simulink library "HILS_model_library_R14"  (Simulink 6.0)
undefined symbols (not defined in the file or in its folder): hilsmdl
libraries: simulink x47, simulink_extras x9, HILS_model_library x3
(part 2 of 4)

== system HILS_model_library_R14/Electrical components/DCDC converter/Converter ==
  ctrl : Inport
  elec in [V] : Inport  Port=2
  elec fb in [A] : Inport  Port=3
  Bus Creator : BusCreator  Inputs=1
  Bus Creator1 : BusCreator  Inputs=2
  Bus Creator5 : BusCreator  Inputs=1
  Bus Selector1 : BusSelector  OutputSignals=phys_current_A
  Bus Selector2 : BusSelector  OutputSignals=Dcdc_ctrl_Rt
  Bus Selector5 : BusSelector  OutputSignals=phys_voltage_V
  Gain : Gain
  Gain1 : Gain
  Memory : Memory  Orientation=left
  Product : Product
  Product1 : Product  Inputs=3
  Sensor : Outport
  elec out [V] : Outport  Port=2
  elec fb out [A] : Outport  Port=3
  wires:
  Bus Creator1/1 -> Sensor/1
  Bus Creator/1 -> elec out [V]/1
  elec in [V]/1 -> Bus Selector5/1
  Bus Creator5/1 -> elec fb out [A]/1
  elec fb in [A]/1 -> Bus Selector1/1
  ctrl/1 -> Bus Selector2/1
  Product/1 -> Bus Creator/1, Gain/1  "phys_voltage_V"
  Product1/1 -> Memory/1, Bus Creator5/1  "phys_current_A"
  Bus Selector1/1 -> Product1/2  "<phys_current_A>"
  Bus Selector5/1 -> Gain1/1, Product/2  "<phys_voltage_V>"
  Bus Selector2/1 -> Product1/1, Product/1  "<Dcdc_ctrl_Rt>"
  Gain/1 -> Bus Creator1/2  "voltage_out"
  Gain1/1 -> Bus Creator1/1  "voltage_in"
  ? -> Product1/3
  Memory/1 -> ?

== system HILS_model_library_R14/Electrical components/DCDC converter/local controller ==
  cmd : Inport
  sensor in : Inport  Port=2
  Bus Creator1 : BusCreator  Inputs=1
  Bus Creator2 : BusCreator  Inputs=1
  Bus Selector1 : BusSelector  OutputSignals=Dcdc_uReq_V
  Bus Selector2 : BusSelector  OutputSignals=voltage_in,voltage_out
  Gain : Gain
  Product : Product  Inputs=*/
  sensor out : Outport
  ctrl : Outport  Port=2
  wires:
  Bus Creator1/1 -> ctrl/1
  sensor in/1 -> Bus Selector2/1
  cmd/1 -> Bus Selector1/1
  Bus Creator2/1 -> sensor out/1  "Dcdc"
  Bus Selector2/1 -> Product/2  "<voltage_in>"
  Bus Selector2/2 -> Gain/1  "<voltage_out>"
  Gain/1 -> Bus Creator2/1  "Dcdc_uAct_V"
  Bus Selector1/1 -> Product/1  "<Dcdc_uReq_V>"
  Product/1 -> Bus Creator1/1  "Dcdc_ctrl_Rt"

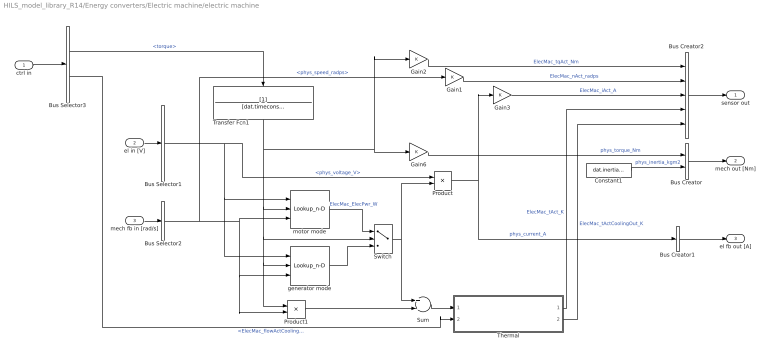
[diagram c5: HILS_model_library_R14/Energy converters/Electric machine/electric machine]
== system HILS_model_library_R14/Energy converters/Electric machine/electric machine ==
  ctrl in : Inport
  el in [V] : Inport  Port=2
  mech fb in [rad/s] : Inport  Port=3
  Bus Creator : BusCreator  Inputs=2
  Bus Creator1 : BusCreator  Inputs=1
  Bus Creator2 : BusCreator  Inputs=5
  Bus Selector1 : BusSelector  OutputSignals=phys_voltage_V
  Bus Selector2 : BusSelector  OutputSignals=phys_speed_radps
  Bus Selector3 : BusSelector  OutputSignals=torque,ElecMac_flowActCooling_kgps
  Constant1 : Constant  Value=dat.inertia.value
  Gain{1..3,6} (4 alike) : Gain
  Product : Product  Inputs=/*
  Product1 : Product  Inputs=**
  Sum : Sum  Inputs=+-
  Switch : Switch
  Thermal : Subsystem
  Transfer Fcn1 : TransferFcn  Orientation=down  Denominator=[dat.timeconstant.value 1]
  generator mode : Lookup_n-D  NumberOfTableDimensions=3  BreakpointsForDimension1=dat.elecpowmap.generator.voltage.vec  BreakpointsForDimension2=dat.elecpowmap.generator.torque.vec  BreakpointsForDimension3=dat.elecpowmap.generator.speed.vec  Table=dat.elecpowmap.generator.elecpow.map  ExtrapMethod=None - Clip
  motor mode : Lookup_n-D  NumberOfTableDimensions=3  BreakpointsForDimension1=dat.elecpowmap.motor.voltage.vec  BreakpointsForDimension2=dat.elecpowmap.motor.torque.vec  BreakpointsForDimension3=dat.elecpowmap.motor.speed.vec  Table=dat.elecpowmap.motor.elecpow.map  ExtrapMethod=None - Clip
  sensor out : Outport
  mech out [Nm] : Outport  Port=2
  el fb out [A] : Outport  Port=3
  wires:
  Sum/1 -> Thermal/1(Total power loss)
  Product1/1 -> Sum/2
  Thermal/1(Machine temperature[K]) -> Bus Creator2/4  "ElecMac_tAct_K"
  Gain6/1 -> Bus Creator/1  "phys_torque_Nm"
  Gain2/1 -> Bus Creator2/1  "ElecMac_tqAct_Nm"
  Gain1/1 -> Bus Creator2/2  "ElecMac_nAct_radps"
  Gain3/1 -> Bus Creator2/3  "ElecMac_iAct_A"
  Product/1 -> Gain3/1, Bus Creator1/1  "phys_current_A"
  Bus Selector3/1 -> Transfer Fcn1/1  "<torque>"
  Constant1/1 -> Bus Creator/2  "phys_inertia_kgm2"
  Bus Creator2/1 -> sensor out/1
  Bus Selector2/1 -> Gain1/1, Product1/2, generator mode/3, motor mode/3  "<phys_speed_radps>"
  ctrl in/1 -> Bus Selector3/1
  mech fb in [rad/s]/1 -> Bus Selector2/1
  el in [V]/1 -> Bus Selector1/1
  Bus Creator/1 -> mech out [Nm]/1
  Bus Creator1/1 -> el fb out [A]/1
  motor mode/1 -> Switch/1  "ElecMac_ElecPwr_W"
  generator mode/1 -> Switch/3
  Switch/1 -> Product/2, Sum/1
  Bus Selector1/1 -> Product/1, motor mode/1, generator mode/1  "<phys_voltage_V>"
  Transfer Fcn1/1 -> Gain2/1, Gain6/1, Product1/1, generator mode/2, Switch/2, motor mode/2
  Bus Selector3/2 -> Thermal/2(Massflow cooling fluid)  "<ElecMac_flowActCooling_kgps>"
  Thermal/2(Fluid outlet temperature[K]) -> Bus Creator2/5  "ElecMac_tActCoolingOut_K"

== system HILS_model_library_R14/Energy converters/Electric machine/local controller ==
  cmd in : Inport
  sensor in : Inport  Port=2
  Bus Creator2 : BusCreator
  Bus Selector1 : BusSelector  OutputSignals=ElecMac_nReq_radps,ElecMac_flgReqSwitch_B,ElecMac_tqReq_Nm,ElecMac_flowActCooling_kgps
  Bus Selector3 : BusSelector  OutputSignals=ElecMac_tqAct_Nm,ElecMac_nAct_radps,ElecMac_iAct_A,ElecMac_tAct_K
  Bus Creator : BusCreator  Inputs=2
  Compare To Zero : simulink/Logic and Bit Operations/Compare To Zero  relop=>  LogicOutDataTypeMode=uint8  ZeroCross=off
  Max torque : Lookup  InputValues=dat.maxtorque.speed.vec  OutputValues=dat.maxtorque.torque.vec  LookUpMeth=Interpolation-Use End Values
  Min torque : Lookup  InputValues=dat.mintorque.speed.vec  OutputValues=dat.mintorque.torque.vec  LookUpMeth=Interpolation-Use End Values
  PI controller : Subsystem
  Product : Product
  Saturation Dynamic : simulink/Discontinuities/Saturation Dynamic  OutDataType=fixdt(1, 16)  OutScaling=2^-10  DoSatur=off
  Switch1 : Switch  Threshold=0.5
  Switch2 : Switch  Threshold=0.5
  sensor out : Outport
  ctrl out : Outport  Port=2
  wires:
  Bus Selector3/4 -> Bus Creator2/4  "<ElecMac_tAct_K>"
  Compare To Zero/1 -> Product/1
  Product/1 -> Switch2/1
  PI controller/1(Ctrl signal) -> Product/2
  Min torque/1 -> Saturation Dynamic/3
  Max torque/1 -> Saturation Dynamic/1
  Switch2/1 -> Saturation Dynamic/2
  Switch1/1 -> PI controller/1(RefSpeed), Switch2/3
  Saturation Dynamic/1 -> Bus Creator/1  "torque"
  Bus Creator/1 -> ctrl out/1
  Bus Selector3/3 -> Bus Creator2/3  "<ElecMac_iAct_A>"
  Bus Selector3/2 -> Min torque/1, Max torque/1, Bus Creator2/2, PI controller/2(ActSpeed)  "<ElecMac_nAct_radps>"
  Bus Selector3/1 -> Bus Creator2/1  "<ElecMac_tqAct_Nm>"
  sensor in/1 -> Bus Selector3/1
  Bus Creator2/1 -> sensor out/1  "ElectricMachine"
  Bus Selector1/3 -> Switch1/3  "<ElecMac_tqReq_Nm>"
  Bus Selector1/2 -> Switch1/2, Switch2/2, PI controller/3(Reset)  "<ElecMac_flgReqSwitch_B>"
  Bus Selector1/1 -> Switch1/1, Compare To Zero/1  "<ElecMac_nReq_radps>"
  cmd in/1 -> Bus Selector1/1
  Bus Selector1/4 -> Bus Creator/2  "<ElecMac_flowActCooling_kgps>"

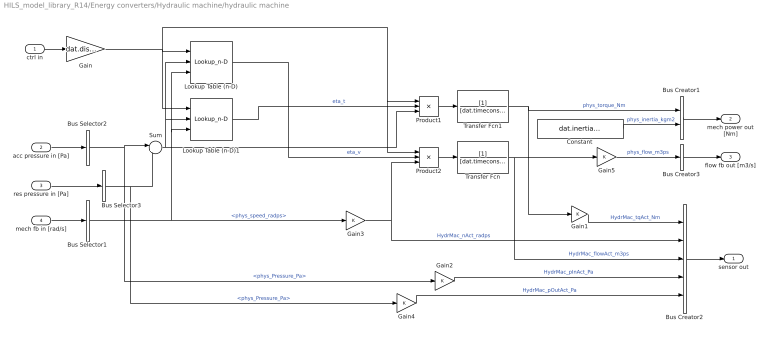
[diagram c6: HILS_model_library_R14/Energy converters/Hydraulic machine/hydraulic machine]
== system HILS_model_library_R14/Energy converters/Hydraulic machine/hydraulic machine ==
  ctrl in : Inport
  acc pressure in [Pa] : Inport  Port=2
  res pressure in [Pa] : Inport  Port=3
  mech fb in [rad/s] : Inport  Port=4
  Bus Creator1 : BusCreator  Inputs=2
  Bus Creator2 : BusCreator  Inputs=5
  Bus Creator3 : BusCreator  Inputs=1
  Bus Selector1 : BusSelector  OutputSignals=phys_speed_radps
  Bus Selector2 : BusSelector  OutputSignals=phys_Pressure_Pa
  Bus Selector3 : BusSelector  OutputSignals=phys_Pressure_Pa
  Constant : Constant  Value=dat.inertia.value
  Gain : Gain  Gain=dat.displacement.value
  Gain{1..5} (5 alike) : Gain
  Lookup Table (n-D) : Lookup_n-D  NumberOfTableDimensions=3  BreakpointsForDimension1=dat.volefficiency.x.vec  BreakpointsForDimension2=dat.volefficiency.pressure.vec  BreakpointsForDimension3=dat.volefficiency.speed.vec  BreakpointsForDimension4=hydraulic_speed_vec_radps  Table=dat.volefficiency.efficiency.map  ExtrapMethod=None - Clip
  Lookup Table (n-D)1 : Lookup_n-D  NumberOfTableDimensions=3  BreakpointsForDimension1=dat.mechefficiency.x.vec  BreakpointsForDimension2=dat.mechefficiency.pressure.vec  BreakpointsForDimension3=dat.mechefficiency.speed.vec  BreakpointsForDimension4=hydraulic_speed_vec_radps  Table=dat.mechefficiency.efficiency.map  ExtrapMethod=None - Clip
  Product1 : Product  Inputs=3
  Product2 : Product  Inputs=3
  Sum : Sum  Inputs=|+-
  Transfer Fcn : TransferFcn  Denominator=[dat.timeconstant.value 1]
  Transfer Fcn1 : TransferFcn  Denominator=[dat.timeconstant.value 1]
  sensor out : Outport
  mech power out [Nm] : Outport  Port=2
  flow fb out [m3/s] : Outport  Port=3
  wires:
  ctrl in/1 -> Gain/1
  Product1/1 -> Transfer Fcn1/1
  Product2/1 -> Transfer Fcn/1
  Gain/1 -> Product1/1, Product2/1, Lookup Table (n-D)/1, Lookup Table (n-D)1/1
  Transfer Fcn/1 -> Bus Creator2/3, Gain5/1  "HydrMac_flowAct_m3ps"
  Transfer Fcn1/1 -> Gain1/1, Bus Creator1/1  "phys_torque_Nm"
  acc pressure in [Pa]/1 -> Bus Selector2/1
  res pressure in [Pa]/1 -> Bus Selector3/1
  Sum/1 -> Product1/3, Lookup Table (n-D)/2, Lookup Table (n-D)1/2
  Bus Creator2/1 -> sensor out/1
  Gain3/1 -> Bus Creator2/2, Product2/3  "HydrMac_nAct_radps"
  Constant/1 -> Bus Creator1/2  "phys_inertia_kgm2"
  Bus Creator1/1 -> mech power out [Nm]/1
  mech fb in [rad/s]/1 -> Bus Selector1/1
  Bus Selector1/1 -> Gain3/1, Lookup Table (n-D)/3, Lookup Table (n-D)1/3  "<phys_speed_radps>"
  Lookup Table (n-D)1/1 -> Product1/2  "eta_t"
  Bus Creator3/1 -> flow fb out [m3/s]/1
  Gain1/1 -> Bus Creator2/1  "HydrMac_tqAct_Nm"
  Bus Selector2/1 -> Sum/1, Gain2/1  "<phys_Pressure_Pa>"
  Bus Selector3/1 -> Gain4/1, Sum/2  "<phys_Pressure_Pa>"
  Gain2/1 -> Bus Creator2/4  "HydrMac_pInAct_Pa"
  Gain4/1 -> Bus Creator2/5  "HydrMac_pOutAct_Pa"
  Gain5/1 -> Bus Creator3/1  "phys_flow_m3ps"
  Lookup Table (n-D)/1 -> Product2/2  "eta_v"

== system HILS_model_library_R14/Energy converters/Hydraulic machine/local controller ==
  cmd in : Inport
  sensor in : Inport  Port=2
  Bus Creator1 : BusCreator  Inputs=1
  Bus Creator2 : BusCreator  Inputs=5
  Bus Selector1 : BusSelector  OutputSignals=HydrMac_nReq_radps,HydrMac_flgRegSwitch_B,HydrMac_tqReg_Nm
  Bus Selector3 : BusSelector  OutputSignals=HydrMac_tqAct_Nm,HydrMac_nAct_radps,HydrMac_flowAct_m3ps,HydrMac_pInAct_Pa,HydrMac_pOutAct_Pa
  PI controller : Subsystem
  Saturation : Saturate  UpperLimit=1  LowerLimit=-1
  Switch1 : Switch  Threshold=0.5
  Switch2 : Switch  Threshold=0.5
  sensor out : Outport
  ctrl out : Outport  Port=2
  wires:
  cmd in/1 -> Bus Selector1/1
  Bus Selector1/1 -> Switch1/1  "<HydrMac_nReq_radps>"
  Bus Selector1/2 -> Switch2/2, PI controller/3(Reset), Switch1/2  "<HydrMac_flgRegSwitch_B>"
  Bus Selector1/3 -> Switch1/3  "<HydrMac_tqReg_Nm>"
  Bus Creator2/1 -> sensor out/1  "HydrMac"
  sensor in/1 -> Bus Selector3/1
  Bus Selector3/2 -> Bus Creator2/2, Switch2/1  "<HydrMac_nAct_radps>"
  Bus Creator1/1 -> ctrl out/1
  Switch1/1 -> PI controller/1(Ref)
  Bus Selector3/1 -> Bus Creator2/1, Switch2/3  "<HydrMac_tqAct_Nm>"
  Switch2/1 -> PI controller/2(Act)
  PI controller/1(Ctrl signal) -> Saturation/1
  Saturation/1 -> Bus Creator1/1
  Bus Selector3/3 -> Bus Creator2/3  "<HydrMac_flowAct_m3ps>"
  Bus Selector3/4 -> Bus Creator2/4  "<HydrMac_pInAct_Pa>"
  Bus Selector3/5 -> Bus Creator2/5  "<HydrMac_pOutAct_Pa>"

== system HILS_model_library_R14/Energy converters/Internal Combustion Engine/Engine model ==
  ctrl in : Inport
  mech fb in [rad/s] : Inport  Port=2
  Bus Creator : BusCreator  Inputs=2
  Bus Creator2 : BusCreator  Inputs=5
  Bus Selector2 : BusSelector  OutputSignals=phys_speed_radps
  Bus Selector3 : BusSelector  OutputSignals=Eng_tqIndReq_Nm,Eng_flgFuelCut_B,Eng_flgOnOff_B,Eng_flgStrtReq_B,Eng_flgExhaustBrake
  Constant1 : Constant  Value=dat.inertia.value
  Engine brake : Lookup  InputValues=dat.exhaustbrake.speed.vec  OutputValues=dat.exhaustbrake.brake.vec  LookUpMeth=Interpolation-Use End Values
  Friction map : Lookup  InputValues=dat.friction.speed.vec  OutputValues=dat.friction.friction.vec  LookUpMeth=Interpolation-Use End Values
  Memory : Memory
  Product : Product
  Product1 : Product  Inputs=3
  Sum1 : Sum
  Sum2 : Sum
  Thermal model ICE : Subsystem
  Torque model1 : Subsystem
  radps2rpm1 : Gain
  radps2rpm2 : Gain
  sensor out : Outport
  mech power out [Nm] : Outport  Port=2
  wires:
  Bus Selector3/4 -> Torque model1/3(starter motor)  "<Eng_flgStrtReq_B>"
  Bus Selector3/3 -> Product1/3  "<Eng_flgOnOff_B>"
  Memory/1 -> Thermal model ICE/2(Eng speed), radps2rpm2/1, Torque model1/2(speed rps), Engine brake/1, Friction map/1
  Bus Creator/1 -> mech power out [Nm]/1
  mech fb in [rad/s]/1 -> Bus Selector2/1
  ctrl in/1 -> Bus Selector3/1
  Bus Selector2/1 -> Memory/1  "<phys_speed_radps>"
  Bus Creator2/1 -> sensor out/1
  Constant1/1 -> Bus Creator/2  "phys_inertia_kgm2"
  Friction map/1 -> Sum2/2  "Eng_tqFrictionAct_Nm"
  Engine brake/1 -> Product/2
  Product/1 -> Sum1/2  "Eng_tqExhaustBrakeAct_Nm"
  Bus Selector3/1 -> Product1/1  "<Eng_tqIndReq_Nm>"
  Bus Selector3/5 -> Product/1  "<Eng_flgExhaustBrake>"
  radps2rpm1/1 -> Bus Creator2/1  "Eng_tqCrkSftAct_Nm"
  radps2rpm2/1 -> Bus Creator2/4  "Eng_nAct_radps"
  Sum1/1 -> Thermal model ICE/1(Torque ICE), radps2rpm1/1, Bus Creator/1  "phys_torque_Nm"
  Thermal model ICE/2(temperature oil [K]) -> Bus Creator2/3  "Eng_tOilAct_K"
  Thermal model ICE/1(temperature cooling fluid [K]) -> Bus Creator2/2  "Eng_tCoolantAct_K"
  Bus Selector3/2 -> Product1/2  "<Eng_flgFuelCut_B>"
  Product1/1 -> Bus Creator2/5, Torque model1/1(Torque in)  "Eng_tqIndAct_Nm"
  Torque model1/1(Torque out) -> Sum2/1
  Sum2/1 -> Sum1/1

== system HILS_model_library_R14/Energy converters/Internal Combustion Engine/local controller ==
  cmd in : Inport
  sensor in : Inport  Port=2
  Bus Creator1 : BusCreator  Inputs=5
  Bus Creator2 : BusCreator
  Bus Selector1 : BusSelector  OutputSignals=Eng_nReq_radps,Eng_flgReqSwitch_B,Eng_tqReq_Nm,Eng_flgFuelCut_B,Eng_flgExhaustBrake,Eng_flgOnOff_B,Eng_flgStrtReq_B
  Bus Selector3 : BusSelector  OutputSignals=Eng_nAct_radps,Eng_tqCrkSftAct_Nm,Eng_tqIndAct_Nm,Eng_tOilAct_K
  Speed controller : Subsystem
  Switch3 : Switch  Threshold=0.5
  Torque Limit : Subsystem
  Torque controller : Subsystem
  sensor : Outport
  ctrl out : Outport  Port=2
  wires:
  Bus Selector1/7 -> Bus Creator1/5  "<Eng_flgStrtReq_B>"
  Bus Selector1/6 -> Bus Creator1/4  "<Eng_flgOnOff_B>"
  cmd in/1 -> Bus Selector1/1
  Bus Selector1/1 -> Speed controller/1(RefSpeed)  "<Eng_nReq_radps>"
  Bus Selector1/2 -> Speed controller/3(Reset), Switch3/2  "<Eng_flgReqSwitch_B>"
  Bus Selector1/3 -> Torque controller/1(RefTorque)  "<Eng_tqReq_Nm>"
  Bus Creator2/1 -> sensor/1  "Engine"
  sensor in/1 -> Bus Selector3/1
  Bus Selector3/1 -> Torque controller/2(ActSpeed), Speed controller/2(ActSpeed), Torque Limit/2(ActSpeed), Bus Creator2/1  "<Eng_nAct_radps>"
  Bus Selector3/2 -> Bus Creator2/2  "<Eng_tqCrkSftAct_Nm>"
  Bus Creator1/1 -> ctrl out/1
  Speed controller/1(ctrl signal) -> Switch3/1
  Torque Limit/1(LimitTorqueDemand) -> Bus Creator1/1
  Switch3/1 -> Torque Limit/1(TorqueDemand)
  Torque controller/1(TotalTorqueRef) -> Switch3/3
  Bus Selector3/3 -> Bus Creator2/3  "<Eng_tqIndAct_Nm>"
  Bus Selector3/4 -> Bus Creator2/4  "<Eng_tOilAct_K>"
  Bus Selector1/5 -> Bus Creator1/3  "<Eng_flgExhaustBrake>"
  Bus Selector1/4 -> Bus Creator1/2  "<Eng_flgFuelCut_B>"

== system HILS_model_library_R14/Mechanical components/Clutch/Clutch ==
  ctrl : Inport
  mech in [Nm] : Inport  Port=2
  mech fb in [rad/s] : Inport  Port=3
  Bus Creator : BusCreator  Inputs=2
  Bus Creator1 : BusCreator  Inputs=1
  Bus Creator5 : BusCreator  Inputs=1
  Bus Selector1 : BusSelector  OutputSignals=phys_speed_radps
  Bus Selector2 : BusSelector  OutputSignals=Clu_ratReq_Rt
  Bus Selector5 : BusSelector  OutputSignals=phys_torque_Nm,phys_inertia_kgm2
  Clutch max  torque [Nm] : Constant  Value=dat.maxtorque.value
  Clutch1 : Subsystem
  Data Type Conversion : DataTypeConversion
  Product : Product
  Saturation : Saturate  UpperLimit=1  LowerLimit=0
  Transfer Fcn : TransferFcn  Denominator=[dat.actuator.timeconstant.value 1]
  sensor out : Outport
  mech out [Nm] : Outport  Port=2
  mech fb out [rad/s] : Outport  Port=3
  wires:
  Transfer Fcn/1 -> Clutch1/1(T_reqClu)
  Product/1 -> Transfer Fcn/1
  Saturation/1 -> Product/1
  Clutch max  torque [Nm]/1 -> Clutch1/5(Maxtorque), Product/2
  Bus Selector2/1 -> Saturation/1  "<Clu_ratReq_Rt>"
  Bus Selector1/1 -> Clutch1/4(w_down)  "<phys_speed_radps>"
  Clutch1/3(w_up) -> Bus Creator5/1  "phys_speed_radps"
  Clutch1/4(B_cluLock) -> Data Type Conversion/1
  Clutch1/1(T_out) -> Bus Creator/1  "phys_torque_Nm"
  ctrl/1 -> Bus Selector2/1
  Bus Creator1/1 -> sensor out/1  "Clutch"
  Bus Selector5/2 -> Clutch1/3(J_in)  "<phys_inertia_kgm2>"
  Bus Selector5/1 -> Clutch1/2(T_in)  "<phys_torque_Nm>"
  Data Type Conversion/1 -> Bus Creator1/1  "Clu_flgConnected_B"
  mech fb in [rad/s]/1 -> Bus Selector1/1
  Bus Creator5/1 -> mech fb out [rad/s]/1
  mech in [Nm]/1 -> Bus Selector5/1
  Bus Creator/1 -> mech out [Nm]/1
  Clutch1/2(J_out) -> Bus Creator/2  "phys_inertia_kgm2"

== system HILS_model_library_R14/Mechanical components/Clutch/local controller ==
  cmd in : Inport
  sensor in : Inport  Port=2
  sensor : Outport
  ctrl : Outport  Port=2
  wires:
  cmd in/1 -> ctrl/1
  sensor in/1 -> sensor/1

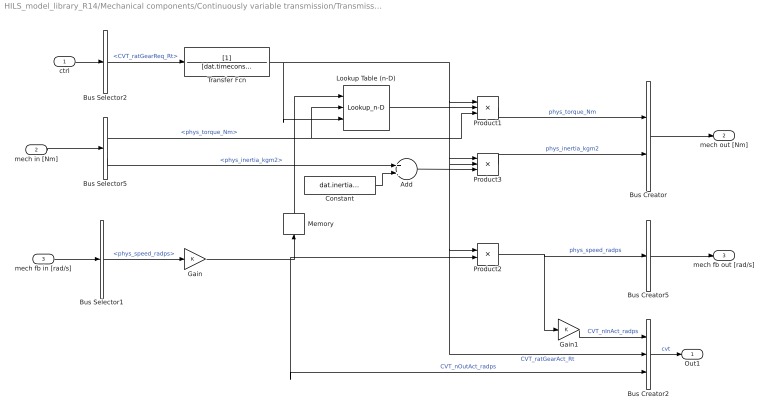
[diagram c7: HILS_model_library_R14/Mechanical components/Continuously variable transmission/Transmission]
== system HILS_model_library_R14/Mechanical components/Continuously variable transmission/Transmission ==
  ctrl : Inport
  mech in [Nm] : Inport  Port=2
  mech fb in [rad/s] : Inport  Port=3
  Add : Sum
  Bus Creator : BusCreator  Inputs=2
  Bus Creator2 : BusCreator  Inputs=3
  Bus Creator5 : BusCreator  Inputs=1
  Bus Selector1 : BusSelector  OutputSignals=phys_speed_radps
  Bus Selector2 : BusSelector  OutputSignals=CVT_ratGearReq_Rt
  Bus Selector5 : BusSelector  OutputSignals=phys_torque_Nm,phys_inertia_kgm2
  Constant : Constant  Value=dat.inertia.value
  Gain : Gain
  Gain1 : Gain
  Lookup Table (n-D) : Lookup_n-D  NumberOfTableDimensions=3  BreakpointsForDimension1=dat.mechefficiency.speed.vec  BreakpointsForDimension2=dat.mechefficiency.torque.vec  BreakpointsForDimension3=dat.mechefficiency.ratio.vec  Table=dat.mechefficiency.efficiency.map  ExtrapMethod=None - Clip
  Memory : Memory  Orientation=up
  Product1 : Product  Inputs=3
  Product2 : Product
  Product3 : Product  Inputs=3
  Transfer Fcn : TransferFcn  Denominator=[dat.timeconstant.value 1]
  Out1 : Outport
  mech out [Nm] : Outport  Port=2
  mech fb out [rad/s] : Outport  Port=3
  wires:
  Bus Selector1/1 -> Gain/1  "<phys_speed_radps>"
  Bus Creator2/1 -> Out1/1  "cvt"
  Bus Creator/1 -> mech out [Nm]/1
  mech in [Nm]/1 -> Bus Selector5/1
  Bus Creator5/1 -> mech fb out [rad/s]/1
  mech fb in [rad/s]/1 -> Bus Selector1/1
  ctrl/1 -> Bus Selector2/1
  Gain1/1 -> Bus Creator2/1  "CVT_nInAct_radps"
  Bus Selector2/1 -> Transfer Fcn/1  "<CVT_ratGearReq_Rt>"
  Product1/1 -> Bus Creator/1  "phys_torque_Nm"
  Product2/1 -> Gain1/1, Bus Creator5/1  "phys_speed_radps"
  Gain/1 -> Memory/1, Product2/2, Bus Creator2/3  "CVT_nOutAct_radps"
  Bus Selector5/1 -> Product1/3, Lookup Table (n-D)/2  "<phys_torque_Nm>"
  Lookup Table (n-D)/1 -> Product1/2
  Bus Selector5/2 -> Add/1  "<phys_inertia_kgm2>"
  Product3/1 -> Bus Creator/2  "phys_inertia_kgm2"
  Add/1 -> Product3/3
  Constant/1 -> Add/2
  Memory/1 -> Lookup Table (n-D)/1
  Transfer Fcn/1 -> Lookup Table (n-D)/3, Product3/2, Product2/1, Bus Creator2/2, Product3/1, Product1/1  "CVT_ratGearAct_Rt"

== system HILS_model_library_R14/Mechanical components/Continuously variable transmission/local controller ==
  cmd : Inport
  sensor in : Inport  Port=2
  Bus Creator1 : BusCreator  Inputs=1
  Bus Creator2 : BusCreator  Inputs=3
  Bus Selector1 : BusSelector  OutputSignals=CVT_ratGearReq_Rt
  Bus Selector2 : BusSelector  OutputSignals=CVT_ratGearAct_Rt,CVT_nInAct_radps,CVT_nOutAct_radps
  sensor out : Outport
  ctrl : Outport  Port=2
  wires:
  Bus Creator1/1 -> ctrl/1
  sensor in/1 -> Bus Selector2/1
  cmd/1 -> Bus Selector1/1
  Bus Creator2/1 -> sensor out/1  "Transmission"
  Bus Selector1/1 -> Bus Creator1/1  "<CVT_ratGearReq_Rt>"
  Bus Selector2/2 -> Bus Creator2/2  "<CVT_nInAct_radps>"
  Bus Selector2/3 -> Bus Creator2/3  "<CVT_nOutAct_radps>"
  Bus Selector2/1 -> Bus Creator2/1  "<CVT_ratGearAct_Rt>"

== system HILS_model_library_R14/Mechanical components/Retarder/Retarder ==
  ctrl : Inport
  mech in [Nm] : Inport  Port=2
  mech fb in [rad/s] : Inport  Port=3
  1-D Lookup Table : Lookup_n-D  NumberOfTableDimensions=1  BreakpointsForDimension1=dat.braketorque.speed.vec  Table=dat.braketorque.torque.vec  ExtrapMethod=None - Clip
  Add : Sum
  Bus Creator : BusCreator  Inputs=2
  Bus Creator1 : BusCreator  Inputs=2
  Bus Creator5 : BusCreator  Inputs=1
  Bus Selector1 : BusSelector  OutputSignals=phys_speed_radps
  Bus Selector2 : BusSelector  OutputSignals=Ret_flgRetBrake
  Bus Selector5 : BusSelector  OutputSignals=phys_torque_Nm,phys_inertia_kgm2
  Constant : Constant  Value=dat.inertia.value
  Gain1 : Gain
  Gain2 : Gain
  Product1 : Product
  Sum : Sum  Inputs=|++
  Out1 : Outport
  mech out [Nm] : Outport  Port=2
  mech fb out [rad/s] : Outport  Port=3
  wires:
  Bus Selector5/2 -> Add/1  "<phys_inertia_kgm2>"
  Sum/1 -> Bus Creator/1, Gain2/1  "phys_torque_Nm"
  Bus Selector2/1 -> Product1/1  "<Ret_flgRetBrake>"
  Gain1/1 -> Bus Creator1/2  "Ret_tqBrkAct_Nm"
  ctrl/1 -> Bus Selector2/1
  mech fb in [rad/s]/1 -> Bus Selector1/1
  Bus Creator5/1 -> mech fb out [rad/s]/1
  mech in [Nm]/1 -> Bus Selector5/1
  Bus Creator/1 -> mech out [Nm]/1
  Bus Creator1/1 -> Out1/1
  Bus Selector1/1 -> 1-D Lookup Table/1, Bus Creator5/1  "<phys_speed_radps>"
  Bus Selector5/1 -> Sum/1  "<phys_torque_Nm>"
  Gain2/1 -> Bus Creator1/1  "Ret_tqAct_Nm"
  1-D Lookup Table/1 -> Product1/2
  Product1/1 -> Gain1/1, Sum/2
  Constant/1 -> Add/2
  Add/1 -> Bus Creator/2  "phys_inertia_kgm2"

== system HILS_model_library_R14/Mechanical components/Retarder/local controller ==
  cmd : Inport
  sensor in : Inport  Port=2
  Bus Creator1 : BusCreator  Inputs=1
  Bus Creator2 : BusCreator  Inputs=2
  Bus Selector1 : BusSelector  OutputSignals=Ret_flgRetBrake
  Bus Selector2 : BusSelector  OutputSignals=Ret_tqAct_Nm,Ret_tqBrkAct_Nm
  sensor out : Outport
  ctrl : Outport  Port=2
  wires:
  Bus Selector2/2 -> Bus Creator2/2  "<Ret_tqBrkAct_Nm>"
  Bus Creator2/1 -> sensor out/1  "Retarder"
  cmd/1 -> Bus Selector1/1
  sensor in/1 -> Bus Selector2/1
  Bus Creator1/1 -> ctrl/1
  Bus Selector1/1 -> Bus Creator1/1  "<Ret_flgRetBrake>"
  Bus Selector2/1 -> Bus Creator2/1  "<Ret_tqAct_Nm>"

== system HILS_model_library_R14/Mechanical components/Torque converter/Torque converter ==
  ctrl : Inport
  mech in [Nm] : Inport  Port=2
  mech fb in [rad/s] : Inport  Port=3
  Bus Creator1 : BusCreator
  Bus Creator2 : BusCreator  Inputs=2
  Bus Creator3 : BusCreator  Inputs=1
  Bus Selector3 : BusSelector  OutputSignals=phys_inertia_kgm2,phys_torque_Nm
  Bus Selector4 : BusSelector  OutputSignals=phys_speed_radps
  Bus Selector6 : BusSelector  OutputSignals=TC_flgLockUp_B
  Constant : Constant  Value=dat.clutch.maxtorque.value
  Data Type Conversion : DataTypeConversion
  Gain : Gain
  Product : Product
  TC : Subsystem
  Transfer Fcn : TransferFcn  Denominator=[dat.clutch.actuator.timeconstant.value 1]
  mech out [Nm] : Outport
  mech fb out [rad/s] : Outport  Port=2
  sensor out : Outport  Port=3
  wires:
  TC/5(sens2) -> Bus Creator1/3  "TC_nTurbineAct_radps"
  TC/4(sens1) -> Bus Creator1/2  "TC_tqTurbineAct_Nm"
  Gain/1 -> Bus Creator1/1  "TC_nPumpAct_radps"
  Product/1 -> TC/1(T_reqClu)
  Constant/1 -> Product/2
  Bus Selector4/1 -> TC/4(w_down)  "<phys_speed_radps>"
  Bus Creator1/1 -> sensor out/1
  TC/6(sens3) -> Bus Creator1/4  "TC_tqPumpAct_Nm"
  Transfer Fcn/1 -> Product/1
  Bus Creator3/1 -> mech fb out [rad/s]/1
  TC/3(w_out) -> Bus Creator3/1, Gain/1  "phys_speed_radps"
  TC/2(J_out) -> Bus Creator2/2  "phys_inertia_kgm2"
  TC/1(T_out) -> Bus Creator2/1  "phys_torque_Nm"
  Bus Selector3/2 -> TC/3(T_in)  "<phys_torque_Nm>"
  Bus Selector3/1 -> TC/2(J_in)  "<phys_inertia_kgm2>"
  Bus Creator2/1 -> mech out [Nm]/1
  ctrl/1 -> Bus Selector6/1
  Bus Selector6/1 -> Data Type Conversion/1  "<TC_flgLockUp_B>"
  mech fb in [rad/s]/1 -> Bus Selector4/1
  mech in [Nm]/1 -> Bus Selector3/1
  Data Type Conversion/1 -> Transfer Fcn/1

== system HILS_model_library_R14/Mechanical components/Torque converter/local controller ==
  cmd : Inport
  sensor in : Inport  Port=2
  Bus Creator1 : BusCreator  Inputs=1
  Bus Creator2 : BusCreator
  Bus Selector1 : BusSelector  OutputSignals=TC_flgLockUp_B
  Bus Selector2 : BusSelector  OutputSignals=TC_nPumpAct_radps,TC_tqTurbineAct_Nm,TC_nTurbineAct_radps,TC_tqPumpAct_Nm
  sensor out : Outport
  ctrl : Outport  Port=2
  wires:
  Bus Selector2/4 -> Bus Creator2/4  "<TC_tqPumpAct_Nm>"
  Bus Selector2/3 -> Bus Creator2/3  "<TC_nTurbineAct_radps>"
  Bus Selector2/2 -> Bus Creator2/2  "<TC_tqTurbineAct_Nm>"
  Bus Selector2/1 -> Bus Creator2/1  "<TC_nPumpAct_radps>"
  Bus Selector1/1 -> Bus Creator1/1  "<TC_flgLockUp_B>"
  Bus Creator1/1 -> ctrl/1
  sensor in/1 -> Bus Selector2/1
  cmd/1 -> Bus Selector1/1
  Bus Creator2/1 -> sensor out/1  "TorqueConverter"

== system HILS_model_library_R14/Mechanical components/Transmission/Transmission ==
  ctrl : Inport
  mech in [Nm] : Inport  Port=2
  mech fb in [rad/s] : Inport  Port=3
  Bus Creator : BusCreator  Inputs=2
  Bus Creator1 : BusCreator
  Bus Creator5 : BusCreator  Inputs=1
  Bus Selector1 : BusSelector  OutputSignals=phys_speed_radps
  Bus Selector2 : BusSelector  OutputSignals=Transm_nrGearReq,Transm_flgCluOpen
  Bus Selector5 : BusSelector  OutputSignals=phys_torque_Nm,phys_inertia_kgm2
  Data Type Conversion : DataTypeConversion
  Gain : Gain
  Gain1 : Gain
  Gain2 : Gain
  torque interupt : Subsystem
  transmission : Subsystem
  Out1 : Outport
  mech out [Nm] : Outport  Port=2
  mech fb out [rad/s] : Outport  Port=3
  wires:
  Gain2/1 -> Bus Creator1/3  "Transm_tqInAct_Nm"
  Data Type Conversion/1 -> Bus Creator1/4  "Transm_flgConnected_B"
  torque interupt/4(B_cluLock) -> Data Type Conversion/1
  Gain1/1 -> Bus Creator1/2  "Transm_nInAct_radps"
  Gain/1 -> Bus Creator1/1, transmission/4(speed)  "Transm_nOutAct_radps"
  torque interupt/3(speed1) -> Gain1/1, Bus Creator5/1
  transmission/3(speed1) -> torque interupt/4(speed)
  torque interupt/2(inertia1) -> transmission/3(inertia)
  torque interupt/1(torque1) -> transmission/2(torque)
  Bus Selector5/1 -> torque interupt/2(torque), Gain2/1  "<phys_torque_Nm>"
  Bus Selector5/2 -> torque interupt/3(inertia)  "<phys_inertia_kgm2>"
  Bus Selector2/1 -> transmission/1(gear)  "<Transm_nrGearReq>"
  Bus Selector2/2 -> torque interupt/1(clutch)  "<Transm_flgCluOpen>"
  ctrl/1 -> Bus Selector2/1
  mech fb in [rad/s]/1 -> Bus Selector1/1
  Bus Creator5/1 -> mech fb out [rad/s]/1
  mech in [Nm]/1 -> Bus Selector5/1
  Bus Creator/1 -> mech out [Nm]/1
  Bus Creator1/1 -> Out1/1  "gearbox"
  transmission/1(torque1) -> Bus Creator/1
  Bus Selector1/1 -> Gain/1  "<phys_speed_radps>"
  transmission/2(inertia1) -> Bus Creator/2

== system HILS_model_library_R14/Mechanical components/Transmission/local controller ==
  cmd : Inport
  sensor in : Inport  Port=2
  Bus Creator1 : BusCreator  Inputs=2
  Bus Creator3 : BusCreator  Inputs=5
  Bus Selector1 : BusSelector  OutputSignals=Transm_nrGearReq
  Bus Selector2 : BusSelector  OutputSignals=Transm_nInAct_radps,Transm_nOutAct_radps,Transm_tqInAct_Nm,Transm_flgConnected_B
  Transport Delay : TransportDelay  DelayTime=dat.timetrqinterrupt.value/2  BufferSize=4096
  clutch operation : Subsystem
  sensor out : Outport
  ctrl : Outport  Port=2
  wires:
  Bus Selector2/4 -> Bus Creator3/5  "<Transm_flgConnected_B>"
  Bus Selector2/3 -> Bus Creator3/4  "<Transm_tqInAct_Nm>"
  Transport Delay/1 -> Bus Creator1/1  "Transm_nrGearReq"
  clutch operation/1(Clutchctrl) -> Bus Creator1/2  "Transm_flgCluOpen"
  clutch operation/2(Actual Gear) -> Bus Creator3/1
  Bus Selector1/1 -> Transport Delay/1, clutch operation/1(Gear)  "<Transm_nrGearReq>"
  Bus Selector2/1 -> Bus Creator3/2  "<Transm_nInAct_radps>"
  Bus Creator3/1 -> sensor out/1  "Transmission"
  cmd/1 -> Bus Selector1/1
  Bus Selector2/2 -> Bus Creator3/3  "<Transm_nOutAct_radps>"
  sensor in/1 -> Bus Selector2/1
  Bus Creator1/1 -> ctrl/1

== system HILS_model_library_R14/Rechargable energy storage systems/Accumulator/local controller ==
  cmd in : Inport
  sensor in : Inport  Port=2
  Bus Creator1 : BusCreator  Inputs=1
  Bus Creator2 : BusCreator  Inputs=2
  Bus Selector2 : BusSelector  OutputSignals=Acc_presAct_Pa,Acc_volGas_Rt
  Ground : Ground
  Model Info : simulink/Model-Wide Utilities/Model Info  InitialBlockCM=None  BlockCM=None  Frame=on  DisplayStringWithTags=|  HorizontalTextAlignment=Left  LeftAlignmentValue=0.02  SourceBlockDiagram=HILS_model_library_R14  TagMaxNumber=20
      | Modified: %<ModifiedDate>
      | 
      | The nodes "cmd in" and "sensor" are fixed.
      | The nodes "sensor in" and "ctrl", however, 
      | may be adjusted arbitrarily since the local controller is 
      | made specifically for a certain component model.
  Model Info1 : simulink/Model-Wide Utilities/Model Info  InitialBlockCM=None  BlockCM=None  Frame=on  DisplayStringWithTags=Your own comments!  HorizontalTextAlignment=Left  LeftAlignmentValue=0.02  SourceBlockDiagram=HILS_model_library_R14  TagMaxNumber=20
  Terminator : Terminator
  sensor : Outport
  ctrl : Outport  Port=2
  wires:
  cmd in/1 -> Terminator/1
  sensor in/1 -> Bus Selector2/1
  Bus Creator2/1 -> sensor/1  "HydrAccumulator"
  Bus Creator1/1 -> ctrl/1
  Ground/1 -> Bus Creator1/1  "empty"
  Bus Selector2/1 -> Bus Creator2/1  "<Acc_presAct_Pa>"
  Bus Selector2/2 -> Bus Creator2/2  "<Acc_volGas_Rt>"

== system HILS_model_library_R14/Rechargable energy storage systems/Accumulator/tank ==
  flow fb in [m3/s]1 : Inport
  flow fb in [m3/s] : Inport  Port=2
  Bus Creator1 : BusCreator  Inputs=2
  Bus Creator2 : BusCreator  Inputs=1
  Bus Selector : BusSelector  OutputSignals=phys_flow_m3ps
  Constant4 : Constant  Value=dat.capacity.value
  Fcn : Fcn  Expr=dat.pressure.precharge.value*(dat.vol.precharge.value/u(1))^dat.gas.adiabaticindex.value
  Fcn1 : Fcn  Expr=-dat.pressure.precharge.value*dat.vol.precharge.value^dat.gas.adiabaticindex.value*(u(1)^(1-dat.gas.adiabaticindex.value)-dat.vol.precharge.value^(1-dat.gas.adiabaticindex.value))/(1-dat.gas.adiabaticindex.value)/1000/3600
  Gain : Gain  Gain=-1
  Gain1 : Gain  Gain=-1
  Integrator : Integrator  InitialCondition=dat.vol.initial.value  LimitOutput=on  UpperSaturationLimit=dat.vol.precharge.value  LowerSaturationLimit=0
  Product1 : Product  Inputs=*/
  Terminator : Terminator
  sensor out : Outport
  pressure out [Pa] : Outport  Port=2
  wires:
  Fcn1/1 -> Product1/1
  Fcn/1 -> Bus Creator2/1, Gain1/1  "phys_pressure_Pa"
  Integrator/1 -> Fcn/1, Fcn1/1
  Bus Creator1/1 -> sensor out/1  "buffer"
  Product1/1 -> Bus Creator1/2  "Acc_volGas_Rt"
  Gain/1 -> Integrator/1
  Constant4/1 -> Product1/2
  Bus Creator2/1 -> pressure out [Pa]/1
  Gain1/1 -> Bus Creator1/1  "Acc_presAct_Pa"
  flow fb in [m3/s]1/1 -> Terminator/1
  flow fb in [m3/s]/1 -> Bus Selector/1
  Bus Selector/1 -> Gain/1  "<phys_flow_m3ps>"

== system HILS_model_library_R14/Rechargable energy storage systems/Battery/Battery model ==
  ctrl in : Inport
  el fb in [A] : Inport  Port=2
  Bus Creator2 : BusCreator  Inputs=5
  Bus Creator3 : BusCreator  Inputs=1
  Bus Selector1 : BusSelector  OutputSignals=Batt_flowActCooling_kgps
  Bus Selector2 : BusSelector  OutputSignals=phys_current_A
  Gain1 : Gain  Gain=1/dat.np.value
  Gain2 : Gain  Gain=dat.ns.value
  Gain3 : Gain  Gain=dat.ns.value*dat.np.value
  Memory : Memory
  Model Info : simulink/Model-Wide Utilities/Model Info  InitialBlockCM=None  BlockCM=None  Frame=on  DisplayStringWithTags=|  HorizontalTextAlignment=Left  LeftAlignmentValue=0.02  SourceBlockDiagram=HILS_model_library_R14  TagMaxNumber=20
      | Modified: %<ModifiedDate>
      | 
      | The nodes "ctrl" and "sensor out" must conform 
      | with the corresponding nodes of the local controller. 
      | The other nodes are fixed.
  Thermal : Subsystem
  single cell model : Subsystem
  sensor out : Outport
  el out [V] : Outport  Port=2
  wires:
  Bus Selector1/1 -> Thermal/2(Massflow cooling fluid)  "<Batt_flowActCooling_kgps>"
  ctrl in/1 -> Bus Selector1/1
  Bus Creator2/1 -> sensor out/1
  Bus Creator3/1 -> el out [V]/1
  el fb in [A]/1 -> Bus Selector2/1
  single cell model/2(voltage) -> Gain2/1
  Gain1/1 -> single cell model/1(current)  "cell_current_A"
  Gain2/1 -> Bus Creator3/1, Bus Creator2/3  "phys_voltage_V"
  single cell model/1(SOC [%]) -> Bus Creator2/2  "phys_soc_proc"
  Bus Selector2/1 -> Bus Creator2/1, Memory/1  "<phys_current_A>"
  Thermal/1(Storage temperature[K]) -> Bus Creator2/4  "Batt_tAct_K"
  single cell model/3(power loss) -> Gain3/1
  Gain3/1 -> Thermal/1(Total power loss)
  Memory/1 -> Gain1/1
  Thermal/2(Fluid outlet temperature[K]) -> Bus Creator2/5  "Batt_tActCoolingOut_K"

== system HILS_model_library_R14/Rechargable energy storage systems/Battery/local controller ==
  cmd in : Inport
  sensor in : Inport  Port=2
  Bus Creator1 : BusCreator  Inputs=1
  Bus Creator2 : BusCreator
  Bus Selector1 : BusSelector  OutputSignals=Batt_flowActCooling_kgps
  Bus Selector2 : BusSelector  OutputSignals=phys_current_A,phys_voltage_V,phys_soc_proc,Batt_tAct_K
  Gain : Gain
  Gain1 : Gain
  Gain2 : Gain  Gain=1/100
  Model Info : simulink/Model-Wide Utilities/Model Info  InitialBlockCM=None  BlockCM=None  Frame=on  DisplayStringWithTags=|  HorizontalTextAlignment=Left  LeftAlignmentValue=0.02  SourceBlockDiagram=HILS_model_library_R14  TagMaxNumber=20
      | Modified: %<ModifiedDate>
      | 
      | The nodes "cmd in" and "sensor" are fixed.
      | The nodes "sensor in" and "ctrl", however, 
      | may be adjusted arbitrarily since the local controller is 
      | made specifically for a certain component model.
  Model Info1 : simulink/Model-Wide Utilities/Model Info  InitialBlockCM=None  BlockCM=None  Frame=on  DisplayStringWithTags=Your own comments!  HorizontalTextAlignment=Left  LeftAlignmentValue=0.02  SourceBlockDiagram=HILS_model_library_R14  TagMaxNumber=20
  sensor : Outport
  ctrl out : Outport  Port=2
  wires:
  Bus Selector1/1 -> Bus Creator1/1  "<Batt_flowActCooling_kgps>"
  Bus Creator1/1 -> ctrl out/1
  Bus Creator2/1 -> sensor/1  "Battery"
  sensor in/1 -> Bus Selector2/1
  Bus Selector2/2 -> Gain1/1  "<phys_voltage_V>"
  Bus Selector2/3 -> Gain2/1  "<phys_soc_proc>"
  cmd in/1 -> Bus Selector1/1
  Gain/1 -> Bus Creator2/1  "Batt_iAct_A"
  Gain1/1 -> Bus Creator2/2  "Batt_uAct_V"
  Gain2/1 -> Bus Creator2/3  "Batt_socAct_Rt"
  Bus Selector2/4 -> Bus Creator2/4  "<Batt_tAct_K>"
  Bus Selector2/1 -> Gain/1  "<phys_current_A>"

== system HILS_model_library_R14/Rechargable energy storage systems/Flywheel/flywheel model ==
  ctrl in : Inport
  mech in [Nm] : Inport  Port=2
  1-D Lookup Table : Lookup_n-D  Orientation=left  NumberOfTableDimensions=1  BreakpointsForDimension1=dat.loss.speed.vec  Table=dat.loss.torqueloss.vec  ExtrapMethod=None - Clip
  Bus Creator : BusCreator  Inputs=1
  Bus Creator2 : BusCreator  Inputs=1
  Bus Selector5 : BusSelector  OutputSignals=phys_torque_Nm,phys_inertia_kgm2
  Constant : Constant  Value=dat.inertia.value
  Gain : Gain
  Integrator : Integrator  LimitOutput=on  UpperSaturationLimit=dat.speedlimit.upper.value  LowerSaturationLimit=dat.speedlimit.lower.value
  Product : Product  Inputs=*/
  Sum : Sum  Inputs=|++
  Sum1 : Sum  Inputs=|+-
  Terminator : Terminator
  sensor out : Outport
  mech fb out [rad/s] : Outport  Port=2
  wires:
  ctrl in/1 -> Terminator/1
  Gain/1 -> Bus Creator2/1  "flywheel_nAct_radps"
  Sum1/1 -> Product/1
  1-D Lookup Table/1 -> Sum1/2
  Sum/1 -> Product/2
  Product/1 -> Integrator/1
  Constant/1 -> Sum/2
  Integrator/1 -> Gain/1, Bus Creator/1, 1-D Lookup Table/1  "phys_speed_radps"
  Bus Selector5/2 -> Sum/1  "<phys_inertia_kgm2>"
  Bus Selector5/1 -> Sum1/1  "<phys_torque_Nm>"
  Bus Creator/1 -> mech fb out [rad/s]/1
  mech in [Nm]/1 -> Bus Selector5/1
  Bus Creator2/1 -> sensor out/1

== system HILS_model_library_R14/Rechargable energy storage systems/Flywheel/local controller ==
  cmd in : Inport
  sensor in : Inport  Port=2
  Bus Creator2 : BusCreator  Inputs=1
  Bus Selector3 : BusSelector  OutputSignals=flywheel_nAct_radps
  Ground : Ground
  Terminator : Terminator
  sensor : Outport
  ctrl out : Outport  Port=2
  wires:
  Bus Selector3/1 -> Bus Creator2/1  "<flywheel_nAct_radps>"
  Ground/1 -> ctrl out/1
  sensor in/1 -> Bus Selector3/1
  Bus Creator2/1 -> sensor/1  "Flywheel"
  cmd in/1 -> Terminator/1

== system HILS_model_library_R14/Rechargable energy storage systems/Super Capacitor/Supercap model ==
  ctrl : Inport
  el fb in [A] : Inport  Port=2
  Bus Creator2 : BusCreator  Inputs=5
  Bus Creator3 : BusCreator  Inputs=1
  Bus Selector1 : BusSelector  OutputSignals=Capa_flowActCooling_kgps
  Bus Selector2 : BusSelector  OutputSignals=phys_current_A
  Gain1 : Gain  Gain=1/dat.np.value
  Gain2 : Gain  Gain=dat.ns.value
  Gain3 : Gain  Gain=dat.ns.value*dat.np.value
  Memory : Memory
  Model Info : simulink/Model-Wide Utilities/Model Info  InitialBlockCM=None  BlockCM=None  Frame=on  DisplayStringWithTags=|  HorizontalTextAlignment=Left  LeftAlignmentValue=0.02  SourceBlockDiagram=HILS_model_library_R14  TagMaxNumber=20
      | Modified: %<ModifiedDate>
      | 
      | The nodes "ctrl" and "sensor out" must conform 
      | with the corresponding nodes of the local controller. 
      | The other nodes are fixed.
  Thermal : Subsystem
  single cell model : Subsystem
  sensor out : Outport
  el out [V] : Outport  Port=2
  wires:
  single cell model/3(power loss) -> Gain3/1
  single cell model/2(voltage) -> Gain2/1
  Memory/1 -> Gain1/1
  Bus Selector2/1 -> Memory/1, Bus Creator2/1  "<phys_current_A>"
  Gain2/1 -> Bus Creator3/1, Bus Creator2/3  "phys_voltage_V"
  Gain1/1 -> single cell model/1(current)  "cell_current_A"
  el fb in [A]/1 -> Bus Selector2/1
  Bus Creator3/1 -> el out [V]/1
  Bus Creator2/1 -> sensor out/1
  ctrl/1 -> Bus Selector1/1
  single cell model/1(SOC [%]) -> Bus Creator2/2  "phys_soc_proc"
  Gain3/1 -> Thermal/1(Total power loss)
  Thermal/1(Storage temperature[K]) -> Bus Creator2/4  "Capa_tAct_K"
  Bus Selector1/1 -> Thermal/2(Massflow cooling fluid)  "<Capa_flowActCooling_kgps>"
  Thermal/2(Fluid outlet temperature[K]) -> Bus Creator2/5  "Capa_tActCoolingOut_K"

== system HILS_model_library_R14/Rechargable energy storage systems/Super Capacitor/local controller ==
  cmd in : Inport
  sensor in : Inport  Port=2
  Bus Creator1 : BusCreator  Inputs=1
  Bus Creator2 : BusCreator
  Bus Selector1 : BusSelector  OutputSignals=Capa_flowActCooling_kgps
  Bus Selector2 : BusSelector  OutputSignals=phys_current_A,phys_voltage_V,phys_soc_proc,Capa_tAct_K
  Gain : Gain
  Gain1 : Gain
  Gain2 : Gain  Gain=1/100
  Model Info : simulink/Model-Wide Utilities/Model Info  InitialBlockCM=None  BlockCM=None  Frame=on  DisplayStringWithTags=|  HorizontalTextAlignment=Left  LeftAlignmentValue=0.02  SourceBlockDiagram=HILS_model_library_R14  TagMaxNumber=20
      | Modified: %<ModifiedDate>
      | 
      | The nodes "cmd in" and "sensor" are fixed.
      | The nodes "sensor in" and "ctrl", however, 
      | may be adjusted arbitrarily since the local controller is 
      | made specifically for a certain component model.
  Model Info1 : simulink/Model-Wide Utilities/Model Info  InitialBlockCM=None  BlockCM=None  Frame=on  DisplayStringWithTags=Your own comments!  HorizontalTextAlignment=Left  LeftAlignmentValue=0.02  SourceBlockDiagram=HILS_model_library_R14  TagMaxNumber=20
  sensor : Outport
  ctrl : Outport  Port=2
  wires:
  Bus Selector2/4 -> Bus Creator2/4  "<Capa_tAct_K>"
  Gain2/1 -> Bus Creator2/3  "Capa_socAct_Rt"
  Gain1/1 -> Bus Creator2/2  "Capa_uAct_V"
  Gain/1 -> Bus Creator2/1  "Capa_iAct_A"
  cmd in/1 -> Bus Selector1/1
  Bus Selector2/3 -> Gain2/1  "<phys_soc_proc>"
  Bus Selector2/2 -> Gain1/1  "<phys_voltage_V>"
  sensor in/1 -> Bus Selector2/1
  Bus Creator2/1 -> sensor/1  "Capacitor"
  Bus Creator1/1 -> ctrl/1
  Bus Selector1/1 -> Bus Creator1/1  "<Capa_flowActCooling_kgps>"
  Bus Selector2/1 -> Gain/1  "<phys_current_A>"

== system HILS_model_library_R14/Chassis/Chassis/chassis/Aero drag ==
  wheel speed : Inport  Orientation=left
  Product1 : Product  Orientation=left  Inputs=***
  aerodynamical drag : Constant  Orientation=left  Value=0.5*hilsmdl.constants.airdensity.value*dat.aero.af.value*dat.aero.cd.value*dat.wheel.radius.value^3
  Tq Aero : Outport  Orientation=left
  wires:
  Product1/1 -> Tq Aero/1
  wheel speed/1 -> Product1/2, Product1/1
  aerodynamical drag/1 -> Product1/3

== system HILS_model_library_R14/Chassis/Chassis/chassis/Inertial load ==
  Pt inertia : Inport  Orientation=up
  mass : Inport  Orientation=up  Port=2
  Constant1 : Constant  Value=dat.wheel.inertia.value
  Sum3 : Sum  Orientation=up  Inputs=+++
  Wheel radius : Gain  Orientation=up  Gain=dat.wheel.radius.value^2
  Total inertia : Outport  Orientation=up
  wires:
  Pt inertia/1 -> Sum3/1
  Sum3/1 -> Total inertia/1
  mass/1 -> Wheel radius/1
  Constant1/1 -> Sum3/2
  Wheel radius/1 -> Sum3/3

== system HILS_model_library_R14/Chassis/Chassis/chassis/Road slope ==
  slope1 : Inport
  Product3 : Product  Inputs=**
  m*g*r : Constant  Value=dat.vehicle.mass.value*hilsmdl.constants.g.value*dat.wheel.radius.value
  slope : Fcn  Expr=sin(u(1))
  Tq slope : Outport
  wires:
  Product3/1 -> Tq slope/1
  slope1/1 -> slope/1
  m*g*r/1 -> Product3/1
  slope/1 -> Product3/2

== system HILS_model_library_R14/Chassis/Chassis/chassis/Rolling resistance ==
  wheel speed : Inport
  slope : Inport  Port=2
  Lookup Table : Lookup  InputValues=[-3e8 -0.1 0.1 3e8]  OutputValues=[-1 -1 1 1]
  Product2 : Product  Inputs=***
  Trigonometric Function : Trigonometry  Operator=cos
  rolling resistance1 : Constant  Value=dat.vehicle.mass.value*hilsmdl.constants.g.value*dat.wheel.rollingres.value*dat.wheel.radius.value
  Tq roll : Outport
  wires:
  Lookup Table/1 -> Product2/1
  Product2/1 -> Tq roll/1
  wheel speed/1 -> Lookup Table/1
  rolling resistance1/1 -> Product2/2
  slope/1 -> Trigonometric Function/1
  Trigonometric Function/1 -> Product2/3

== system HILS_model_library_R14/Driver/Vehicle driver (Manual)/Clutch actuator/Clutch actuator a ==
  Drv_gearReq : Inport
  Clutch locked S-R Flip-Flop : simulink_extras/Flip Flops/S-R Flip-Flop  initial_condition=0
  Clutch locked S-R Flip-Flop1 : simulink_extras/Flip Flops/S-R Flip-Flop  initial_condition=0
  Data Type Conversion1 : DataTypeConversion
  Data Type Conversion2 : DataTypeConversion
  Data Type Conversion4 : DataTypeConversion
  Detect Decrease : simulink/Logic and Bit Operations/Detect Decrease  vinit=0.0
  Detect Increase : simulink/Logic and Bit Operations/Detect Increase  vinit=0.0
  Relational Operator : RelationalOperator  Operator===
  Terminator : Terminator
  Terminator1 : Terminator
  Transport Delay : TransportDelay  DelayTime=dat.clutchtime.value
  DrvReqCluGearDwn : Outport
  DrvReqCluGearUp : Outport  Port=2
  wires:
  Relational Operator/1 -> Data Type Conversion1/1
  Transport Delay/1 -> Relational Operator/2
  Data Type Conversion2/1 -> Clutch locked S-R Flip-Flop1/1
  Detect Decrease/1 -> Data Type Conversion2/1
  Clutch locked S-R Flip-Flop1/2 -> Terminator/1
  Clutch locked S-R Flip-Flop/2 -> Terminator1/1
  Clutch locked S-R Flip-Flop1/1 -> DrvReqCluGearDwn/1
  Drv_gearReq/1 -> Detect Increase/1, Transport Delay/1, Detect Decrease/1, Relational Operator/1
  Detect Increase/1 -> Data Type Conversion4/1
  Clutch locked S-R Flip-Flop/1 -> DrvReqCluGearUp/1
  Data Type Conversion4/1 -> Clutch locked S-R Flip-Flop/1
  Data Type Conversion1/1 -> Clutch locked S-R Flip-Flop1/2, Clutch locked S-R Flip-Flop/2

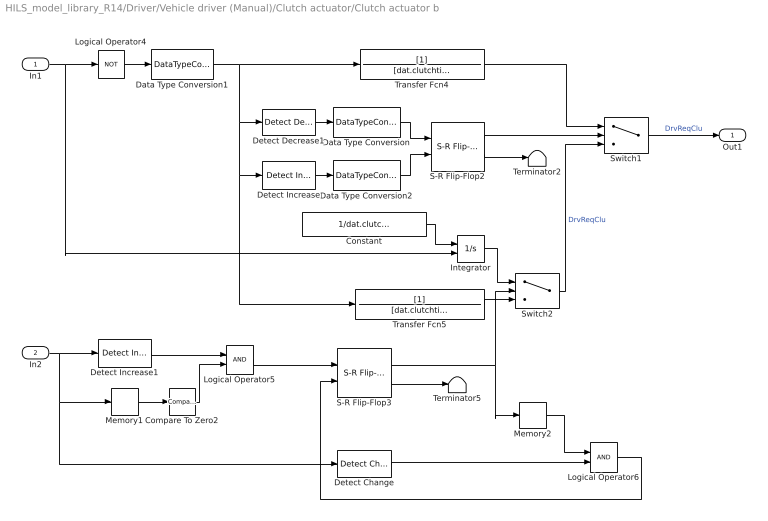
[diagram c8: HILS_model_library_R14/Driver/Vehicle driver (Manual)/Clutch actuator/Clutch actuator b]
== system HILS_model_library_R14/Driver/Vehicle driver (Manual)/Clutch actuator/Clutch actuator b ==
  In1 : Inport
  In2 : Inport  Port=2
  Compare To Zero2 : simulink/Logic and Bit Operations/Compare To Zero  relop===  LogicOutDataTypeMode=boolean
  Constant : Constant  Value=1/dat.clutchtime.driveaway.value
  Data Type Conversion : DataTypeConversion
  Data Type Conversion1 : DataTypeConversion
  Data Type Conversion2 : DataTypeConversion
  Detect Change : simulink/Logic and Bit Operations/Detect Change  vinit=0
  Detect Decrease1 : simulink/Logic and Bit Operations/Detect Decrease  vinit=0.0
  Detect Increase : simulink/Logic and Bit Operations/Detect Increase  vinit=0.0
  Detect Increase1 : simulink/Logic and Bit Operations/Detect Increase  vinit=0.0
  Integrator : Integrator  ExternalReset=either  LimitOutput=on  UpperSaturationLimit=1  LowerSaturationLimit=0
  Logical Operator4 : Logic  Operator=NOT  AllPortsSameDT=off
  Logical Operator5 : Logic  AllPortsSameDT=off
  Logical Operator6 : Logic  AllPortsSameDT=off
  Memory1 : Memory
  Memory2 : Memory
  S-R Flip-Flop2 : simulink_extras/Flip Flops/S-R Flip-Flop  initial_condition=0
  S-R Flip-Flop3 : simulink_extras/Flip Flops/S-R Flip-Flop  initial_condition=0
  Switch1 : Switch  Threshold=1
  Switch2 : Switch  Threshold=1
  Terminator2 : Terminator
  Terminator5 : Terminator
  Transfer Fcn4 : TransferFcn  Denominator=[dat.clutchtime.open.value 1]
  Transfer Fcn5 : TransferFcn  Denominator=[dat.clutchtime.close.value 1]
  Out1 : Outport
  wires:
  Constant/1 -> Integrator/1
  In2/1 -> Memory1/1, Detect Change/1, Detect Increase1/1
  Data Type Conversion1/1 -> Transfer Fcn5/1, Detect Increase/1, Detect Decrease1/1, Transfer Fcn4/1
  Detect Increase/1 -> Data Type Conversion2/1
  Switch1/1 -> Out1/1  "DrvReqClu"
  Transfer Fcn4/1 -> Switch1/1
  In1/1 -> Logical Operator4/1, Integrator/2
  Logical Operator4/1 -> Data Type Conversion1/1
  Detect Decrease1/1 -> Data Type Conversion/1
  Transfer Fcn5/1 -> Switch2/3
  S-R Flip-Flop3/2 -> Terminator5/1
  S-R Flip-Flop3/1 -> Memory2/1, Switch2/2
  Switch2/1 -> Switch1/3  "DrvReqClu"
  S-R Flip-Flop2/1 -> Switch1/2
  S-R Flip-Flop2/2 -> Terminator2/1
  Integrator/1 -> Switch2/1
  Logical Operator5/1 -> S-R Flip-Flop3/1
  Logical Operator6/1 -> S-R Flip-Flop3/2
  Memory2/1 -> Logical Operator6/1
  Detect Increase1/1 -> Logical Operator5/1
  Detect Change/1 -> Logical Operator6/2
  Compare To Zero2/1 -> Logical Operator5/2
  Memory1/1 -> Compare To Zero2/1
  Data Type Conversion/1 -> S-R Flip-Flop2/1
  Data Type Conversion2/1 -> S-R Flip-Flop2/2

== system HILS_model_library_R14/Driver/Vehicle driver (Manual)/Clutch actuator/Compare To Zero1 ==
  u : Inport
  Compare : RelationalOperator  Operator===
  Ground : Ground  DisableCoverage=on
  Signal Specification : SignalSpecification  DisableCoverage=on  Dimensions=1
  y : Outport
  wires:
  Compare/1 -> y/1
  Ground/1 -> Signal Specification/1
  u/1 -> Compare/1
  Signal Specification/1 -> Compare/2

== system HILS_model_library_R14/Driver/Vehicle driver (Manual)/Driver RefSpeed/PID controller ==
  PI reset : Inport
  PI input : Inport  Port=2
  Add : Sum  Inputs=+++
  Derivative : Derivative
  Integrator : Integrator  ExternalReset=rising  UpperSaturationLimit=30  LowerSaturationLimit=0
  Kd : Gain  Gain=dat.controller.d.value
  Ki : Gain  Gain=dat.controller.i.value
  Kp : Gain  Gain=dat.controller.p.value
  Kw : Gain  Orientation=left  Gain=dat.controller.k.value
  Saturation : Saturate  UpperLimit=1  LowerLimit=-1
  Sum1 : Sum  Inputs=|++
  Sum2 : Sum  Orientation=left  Inputs=-+|
  PI output : Outport
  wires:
  Derivative/1 -> Add/2
  Kd/1 -> Derivative/1
  PI input/1 -> Kd/1, Kp/1, Ki/1
  Integrator/1 -> Add/3
  Add/1 -> Saturation/1, Sum2/1
  Saturation/1 -> PI output/1, Sum2/2
  PI reset/1 -> Integrator/2
  Kp/1 -> Add/1
  Ki/1 -> Sum1/1
  Sum1/1 -> Integrator/1
  Sum2/1 -> Kw/1
  Kw/1 -> Sum1/2

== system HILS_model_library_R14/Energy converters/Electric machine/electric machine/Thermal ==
  Total power loss : Inport
  Massflow cooling fluid : Inport  Port=2
  Bus Creator2 : BusCreator  Inputs=2
  Cooling2 : Subsystem
  c2 : Constant  Value=dat.coolingFluid.flowTemp.value
  Machine temperature[K] : Outport
  Fluid outlet temperature[K] : Outport  Port=2
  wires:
  Bus Creator2/1 -> Cooling2/2(cooling inlet)
  c2/1 -> Bus Creator2/2  "temperature [K]"
  Massflow cooling fluid/1 -> Bus Creator2/1  "mass flow [kg/s]"
  Cooling2/1(internal temperature) -> Machine temperature[K]/1  "ElecMac_tAct_K"
  Total power loss/1 -> Cooling2/1(power loss)
  Cooling2/2(fluid outlet temperature) -> Fluid outlet temperature[K]/1  "ElecMac_tActCoolingOut_K"

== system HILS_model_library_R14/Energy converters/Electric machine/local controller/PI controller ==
  RefSpeed : Inport
  ActSpeed : Inport  Port=2
  Reset : Inport  Port=3
  Gain : Gain  Gain=dat.controller.i.value
  Gain2 : Gain  Gain=dat.controller.p.value
  Integrator : Integrator  ExternalReset=either
  Product : Product
  Sum : Sum  Inputs=|+-
  Sum1 : Sum  Inputs=|++
  Ctrl signal : Outport
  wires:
  Sum1/1 -> Ctrl signal/1
  Reset/1 -> Integrator/2, Product/2
  ActSpeed/1 -> Sum/2
  RefSpeed/1 -> Sum/1
  Product/1 -> Integrator/1
  Gain/1 -> Product/1
  Gain2/1 -> Sum1/2
  Integrator/1 -> Sum1/1
  Sum/1 -> Gain2/1, Gain/1
